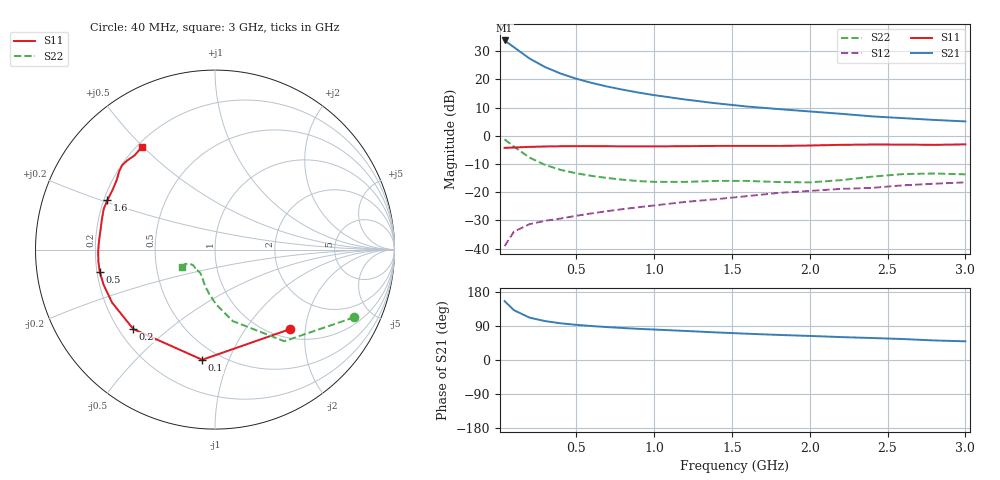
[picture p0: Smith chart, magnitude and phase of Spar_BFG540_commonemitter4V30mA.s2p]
! Filename:  BFG540D.S2P  Version:  3.0
! NXP part #: BFG540  Date: Feb 1992
! Bias condition: Vce=4V, Ic=30mA
! IN LINE PINNING: same data as with cross emitter pinning.
#  MHz  S  MA  R  50
! Freq  S11  S21  S12  S22  !GUM [dB]
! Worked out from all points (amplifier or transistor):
!   21 points, 40 MHz to 3 GHz, reference 50 ohm
!   highest |S21| = 33.8 dB at 40 MHz (marker M1)
!   |S21| within 3 dB of that: start of sweep to 114.9 MHz
!   unconditionally stable (mu >= 1): 791.3 MHz to end of sweep
!   at 300 MHz: K = 0.60, MSG = 27.3 dB, |S12| = -30.2 dB
!   at 1 GHz: K = 1.09, MAG = 17.7 dB, |S12| = -24.7 dB
!   at 3 GHz: K = 1.15, MAG = 8.5 dB, |S12| = -16.5 dB
!   lowest NFmin = 1.70 dB at 900 MHz
!   S11 on the Smith chart (normalised r, x): 40 MHz: 1.18, -1.66; 100 MHz: 0.41, -0.81; 200 MHz: 0.26, -0.38; 500 MHz: 0.21, -0.09; 1.6 GHz: 0.21, +0.21; 3 GHz: 0.22, +0.50
40  0.61 -46.5  49 155.3  0.011 69.0  0.863 -25.9
100  0.618 -96.6  37.16 131.4  0.02 53.2  0.64 -52.9
200  0.635 -135.8  23.44 111.8  0.027 45.2  0.41 -76.1
300  0.645 -152.8  16.53 102.6  0.031 44.8  0.304 -89.0
400  0.651 -162.5  12.68 96.9  0.034 47.7  0.248 -97.6
500  0.654 -169.1  10.28 92.8  0.038 50.2  0.216 -103.9
600  0.653 -174.2  8.647 89.6  0.042 53.4  0.194 -108.7
700  0.651 -178.5  7.455 86.8  0.046 55.3  0.178 -112.6
800  0.649 177.7  6.554 84.4  0.05 57.2  0.166 -116.4
900  0.647 174.1  5.835 82.2  0.054 59.3  0.157 -120.6
1000  0.647 170.6  5.261 80.4  0.058 60.7  0.152 -124.5
1200  0.653 164.6  4.395 76.7  0.067 62.8  0.152 -131.2
1400  0.66 159.9  3.76 72.8  0.075 63.6  0.158 -133.9
1600  0.66 155.3  3.293 69.3  0.085 65.3  0.158 -134.7
1800  0.66 150.1  2.973 66.2  0.097 65.2  0.151 -137.1
2000  0.671 144.7  2.697 63.5  0.105 65.9  0.149 -144.2
2200  0.69 140.6  2.452 60.5  0.114 65.8  0.163 -151.7
2400  0.699 137.7  2.207 58.0  0.119 66.5  0.188 -154.4
2600  0.697 134.6  2.052 55.3  0.132 65.5  0.209 -152.5
2800  0.69 130.4  1.908 51.6  0.141 63.3  0.214 -150.0
3000  0.703 125.3  1.796 49.3  0.149 63.9  0.207 -151.7
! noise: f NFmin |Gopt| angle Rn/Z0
900  1.7  0.312  171  0.11
2000  2.4  0.543  -155  0.12
